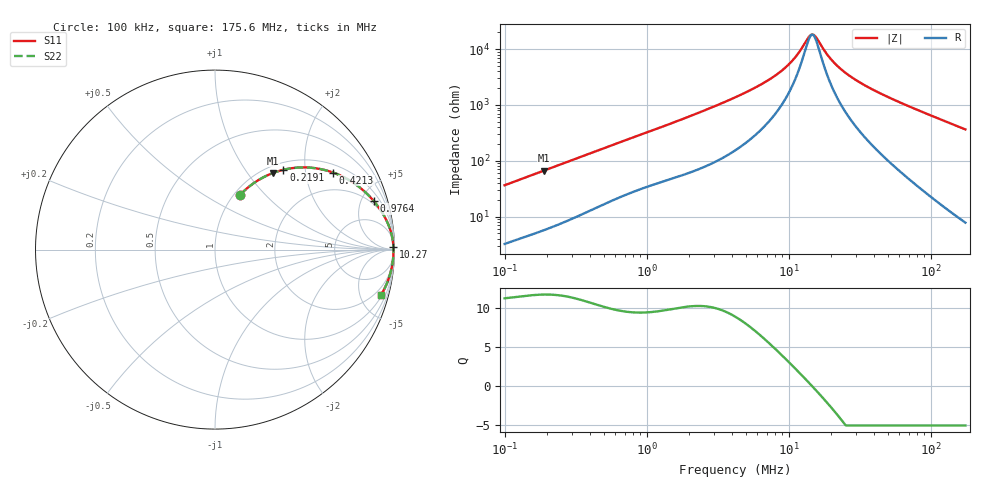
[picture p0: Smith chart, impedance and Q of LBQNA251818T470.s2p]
! LBQNA251818T470  S-PARAMETER MODEL  ( General Type )
! Model Generated by TAIYO YUDEN Corporation (http://www.ty-top.com)
! Version 1.0
! TAIYO YUDEN Control No. 191025NI43SB-FBB
! Copyright(c) 2019 TAIYO YUDEN CO.,LTD. All Rights Reserved.
! Product Description (link to TY-COMPAS)
! https://ds.yuden.co.jp/TYCOMPAS/or/detail?pn=LBQNA251818T470K&u=M
! Products Name : Inductors
! Characteristics :
!  Inductance : 47 uH , SRF(min) : 12 MHz , DC Resistance(max) : 1.235 Ohm
!  Rated Current : Saturation :110 mA , Temp Rise : 270 mA (20 degC)
!  Case Size : 2.5 x 1.8 / 0.098 x 0.071 [mm/inch] , Thickness : 1.8 / 0.071 [mm/inch]
!  (Conditions: Temperature = 25 degC , DC Bias Current/Voltage = 0A / 0V)
! External Node Assignments :
!  1  o---GGG---o  2
! GND o---------o GND
! Frequency Range : 0.1MHz  -  175.64884MHz  [ 402 STEP ]
# MHz S RI R 50
! Freq[MHz].  S11 Real  S11 Imag  S21 Real  S21 Imag  S12 Real  S12 Imag  S22 Real  S22 Imag
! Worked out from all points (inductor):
!   401 points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, 100 kHz to 175.6 MHz, reference 50 ohm
!   read as one part in series: L = 57 uH near 103.8 kHz
!   highest Q = 11.7 at 188.7 kHz (marker M1), where L = 56 uH
!   self-resonance near 14.65 MHz
!   S11 on the Smith chart (normalised r, x): 100 kHz: 1.06, +0.72; 219.1 kHz: 1.13, +1.53; 421.3 kHz: 1.27, +2.86; 976.4 kHz: 1.66, +6.24; 10.27 MHz: open; 175.6 MHz: 1.16, -7.30
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0.1  0.1376 0.3028  0.8624 -0.3028  0.8624 -0.3028  0.1376 0.3028
0.18871  0.3217 0.4263  0.6783 -0.4263  0.6783 -0.4263  0.3217 0.4263
0.219123  0.3815 0.4448  0.6185 -0.4448  0.6185 -0.4448  0.3815 0.4448
0.349525  0.5835 0.4495  0.4165 -0.4495  0.4165 -0.4495  0.5835 0.4495
0.421303  0.6589 0.4289  0.3411 -0.4289  0.3411 -0.4289  0.6589 0.4289
0.635404  0.7928 0.3568  0.2072 -0.3568  0.2072 -0.3568  0.7928 0.3568
0.976375  0.8842 0.2711  0.1158 -0.2711  0.1158 -0.2711  0.8842 0.2711
1.221676  0.9164 0.2294  0.0836 -0.2294  0.0836 -0.2294  0.9164 0.2294
4.270063  0.987 0.0698  0.013 -0.0698  0.013 -0.0698  0.987 0.0698
7.203763  0.9925 0.0348  0.00751 -0.0348  0.00751 -0.0348  0.9925 0.0348
8.683115  0.9934 0.0248  0.00657 -0.0248  0.00657 -0.0248  0.9934 0.0248
10.27259  0.994 0.0165  0.006 -0.0165  0.006 -0.0165  0.994 0.0165
11.70743  0.9943 0.0103  0.0057 -0.0103  0.0057 -0.0103  0.9943 0.0103
13.85051  0.9945 0.00258  0.00547 -0.00258  0.00547 -0.00258  0.9945 0.00258
14.64875  0.9946 2.99e-05  0.00543 -2.99e-05  0.00543 -2.99e-05  0.9946 2.99e-05
15.78509  0.9946 -0.00337  0.0054 0.00337  0.0054 0.00337  0.9946 -0.00337
20.12325  0.9945 -0.0147  0.0055 0.0147  0.0055 0.0147  0.9945 -0.0147
24.25573  0.9942 -0.0239  0.00581 0.0239  0.00581 0.0239  0.9942 -0.0239
33.32052  0.9931 -0.0417  0.00693 0.0417  0.00693 0.0417  0.9931 -0.0417
51.20104  0.9895 -0.0727  0.0105 0.0727  0.0105 0.0727  0.9895 -0.0727
96.62148  0.9735 -0.1436  0.0265 0.1436  0.0265 0.1436  0.9735 -0.1436
175.6488  0.9255 -0.2521  0.0745 0.2521  0.0745 0.2521  0.9255 -0.2521
